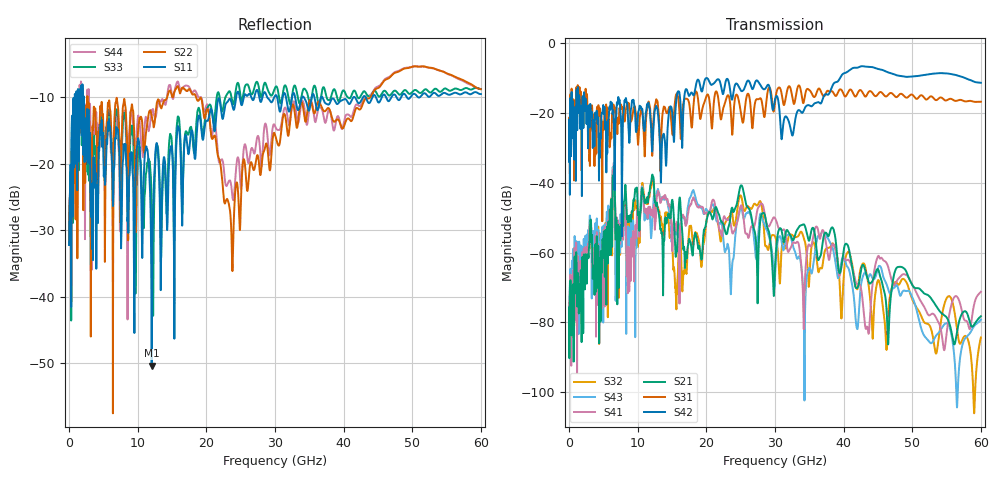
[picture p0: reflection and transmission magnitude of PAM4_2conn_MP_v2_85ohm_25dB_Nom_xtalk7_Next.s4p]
! Info: Touchstone file created by Circ.  Input file=FAB50GbE_2conn_Midplane_Examax_Topo2_v2_85ohm_25dB_Nom.circ
# Hz S RI R 50
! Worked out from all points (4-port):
!   6000 points, 10 MHz to 60 GHz, reference 50 ohm
!   strongest paths, dB at 10 MHz, 15.01 GHz, 30.01 GHz, 45.01 GHz, 60 GHz:
!     S42: -34.0, -19.7, -16.3, -7.5, -11.4
!     S31: -33.7, -25.0, -16.8, -14.6, -16.9
!     S21: -75.8, -45.0, -64.3, -64.8, -78.3
!     S41: -88.9, -58.3, -50.2, -61.1, -71.2
!     S43: -77.5, -54.6, -66.9, -64.5, -79.2
!     S32: -81.1, -56.0, -55.4, -68.0, -84.3
!   lowest |S11| = -50.4 dB at 12.04 GHz (marker M1), VSWR 1.01, Z = 50 - j0.3 ohm
!   |S11| at or under -10 dB: 2.159 GHz to 24.35 GHz (22.19 GHz wide, 167 % of centre); 36.89 GHz to 41.5 GHz (4.615 GHz wide, 11.8 % of centre); 41.56 GHz to 42.85 GHz (1.293 GHz wide, 3.06 % of centre)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
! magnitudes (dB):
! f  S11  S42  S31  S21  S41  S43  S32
! 10 MHz  -32.2  -34.0  -33.7  -75.8  -88.9  -77.5  -81.1
! 6.35 GHz  -23.7  -20.4  -21.8  -40.3  -36.6  -35.7  -39.5
! 12.04 GHz  -50.4  -28.4  -27.4  -38.5  -47.8  -53.8  -40.1
! 15.58 GHz  -18.7  -17.2  -14.9  -60.9  -53.8  -54.7  -73.5
! 24.97 GHz  -10.6  -13.4  -19.1  -41.0  -46.9  -47.4  -43.6
! 43.36 GHz  -10.4  -6.8  -15.0  -66.6  -81.4  -66.7  -66.4
! 60 GHz  -9.6  -11.4  -16.9  -78.3  -71.2  -79.2  -84.3
